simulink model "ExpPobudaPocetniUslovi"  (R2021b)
settings: Solver=ode45  StartTime=0.0  StopTime=0.1  MaxStep=1e-7  RelTol=1e-3  EnableMultiTasking=on
libraries: fl_lib x10, nesl_utility x4, simulink x1

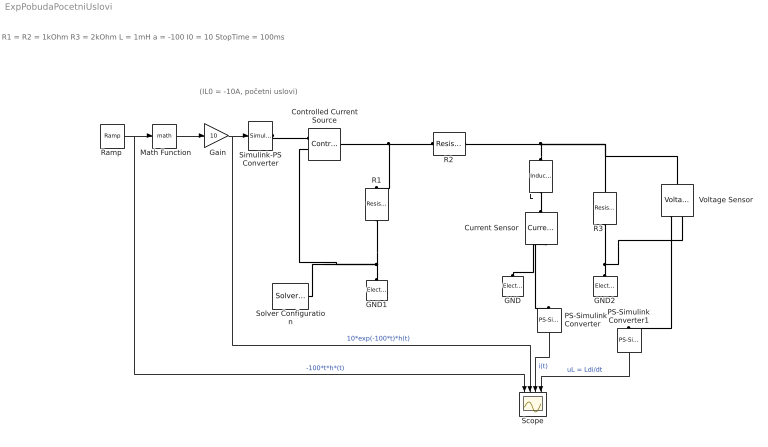
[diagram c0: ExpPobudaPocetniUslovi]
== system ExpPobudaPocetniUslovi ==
  note: (IL0 = -10A, početni uslovi)
  note: R1 = R2 = 1kOhm R3 = 2kOhm L = 1mH a = -100 I0 = 10 StopTime = 100ms
  " Gain" : Gain  Gain=10
  " Math Function" : Math  SignedPower=on
  " Voltage Sensor" : fl_lib/Electrical/Electrical Sensors/Voltage Sensor
  Controlled Current Source : fl_lib/Electrical/Electrical Sources/Controlled Current Source
  "Current Sensor " : fl_lib/Electrical/Electrical Sensors/Current Sensor
  GND : fl_lib/Electrical/Electrical Elements/Electrical Reference
  GND1 : fl_lib/Electrical/Electrical Elements/Electrical Reference
  GND2 : fl_lib/Electrical/Electrical Elements/Electrical Reference
  L : fl_lib/Electrical/Electrical Elements/Inductor  l=1e-3 H  r=0 Ohm  g=0 1/Ohm  i_specify=off  i_priority=None  i=0 A  i_nominal_specify=off  i_nominal_unit=A  i_nominal_value=1  v_specify=off  v_priority=None  v=0 V  v_nominal_specify=off  v_nominal_unit=V  v_nominal_value=1  i_L_specify=on  i_L_priority=High  i_L=-10 A  i_L_nominal_specify=off  i_L_nominal_unit=A  i_L_nominal_value=1
  PS-Simulink Converter : nesl_utility/PS-Simulink Converter  PhysicalDomain=network_engine_domain  SubClassName=ps_output  LeftPortType=input  RightPortType=output  PseudoPeriodic=off  Frequencies=[]  Unit=1  AffineConversion=off
  PS-Simulink Converter1 : nesl_utility/PS-Simulink Converter  PhysicalDomain=network_engine_domain  SubClassName=ps_output  LeftPortType=input  RightPortType=output  PseudoPeriodic=off  Frequencies=[]  Unit=1  AffineConversion=off
  R1 : fl_lib/Electrical/Electrical Elements/Resistor  R=1 kOhm  i_specify=off  i_priority=None  i=0 A  i_nominal_specify=off  i_nominal_unit=A  i_nominal_value=1  v_specify=off  v_priority=None  v=0 V  v_nominal_specify=off  v_nominal_unit=V  v_nominal_value=1
  R2 : fl_lib/Electrical/Electrical Elements/Resistor  R=1 kOhm  i_specify=off  i_priority=None  i=0 A  i_nominal_specify=off  i_nominal_unit=A  i_nominal_value=1  v_specify=off  v_priority=None  v=0 V  v_nominal_specify=off  v_nominal_unit=V  v_nominal_value=1
  R3 : fl_lib/Electrical/Electrical Elements/Resistor  R=2 kOhm  i_specify=off  i_priority=None  i=0 A  i_nominal_specify=off  i_nominal_unit=A  i_nominal_value=1  v_specify=off  v_priority=None  v=0 V  v_nominal_specify=off  v_nominal_unit=V  v_nominal_value=1
  "Ramp " : simulink/Sources/Ramp  slope=-100  start=0  InitialOutput=0
  Scope : Scope  NumInputPorts=4
  Simulink-PS Converter : nesl_utility/Simulink-PS Converter  PhysicalDomain=network_engine_domain  SubClassName=ps_input  LeftPortType=input  RightPortType=output  PseudoPeriodic=off  Frequencies=[]  NoiseDistribution=none  NoiseParameters=[]  Unit=1  AffineConversion=off  FilteringAndDerivatives=zero  SimscapeFilterOrder=1  InputFilterTimeConstant=0.001  UdotUserProvided=1
  Solver Configuration : nesl_utility/Solver Configuration  PhysicalDomain=network_engine_domain  SubClassName=solver  LeftPortType=input  RightPortType=generic  Tones=[]  Harmonics=[]  SimulateNoise=off  Profile=off  UseLocalSampling=off  EnableSwitchedLinearOptims=on  FrequencyDomain=off  UseCCode=off  RelTol=0.001  AbsTol=1e-06  MinStep=1e-09  ToWorkspace=off  RevertToSquareIcSolve=off  NumHomotopyIterations=100  PhasorMode=off  PhasorModeNumHarmonics=1  DoDC=off  ResidualTolerance=1e-09  UseLocalSolver=off  LocalSolverChoice=NE_BACKWARD_EULER_ADVANCER  LocalSolverSampleTime=0.001  DoFixedCost=off  MaxNonlinIter=3  MaxModeIter=2  ComputeImpulses=off  ImpulseIterations=2  LinearAlgebra=Sparse  EquationFormulation=NE_TIME_EF  DelaysMemoryBudget=1024  AutomaticFiltering=on  FilteringTimeConstant=0.001  PartitionStorageMethod=AS_NEEDED  PartitionMemoryBudget=1024  PartitionMethod=FAST
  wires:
  " Math Function"/1 -> " Gain"/1
  "Ramp "/1 -> Scope/1, " Math Function"/1  "-100*t*h*(t)"
  PS-Simulink Converter/1 -> Scope/3  "i(t)"
  " Gain"/1 -> Scope/2, Simulink-PS Converter/1  "10*exp(-100*t)*h(t)"
  PS-Simulink Converter1/1 -> Scope/4  "uL = Ldi/dt"
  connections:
  R2/LConn1 -- R1/LConn1 -- Controlled Current Source/LConn1
  R1/RConn1 -- Solver Configuration/RConn1 -- Controlled Current Source/RConn2 -- GND1/LConn1
  L/LConn1 -- " Voltage Sensor"/LConn1 -- R3/LConn1 -- R2/RConn1
  L/RConn1 -- "Current Sensor "/LConn1
  GND/LConn1 -- "Current Sensor "/RConn2
  "Current Sensor "/RConn1 -- PS-Simulink Converter/LConn1
  GND2/LConn1 -- " Voltage Sensor"/RConn2 -- R3/RConn1
  Simulink-PS Converter/RConn1 -- Controlled Current Source/RConn1
  " Voltage Sensor"/RConn1 -- PS-Simulink Converter1/LConn1
